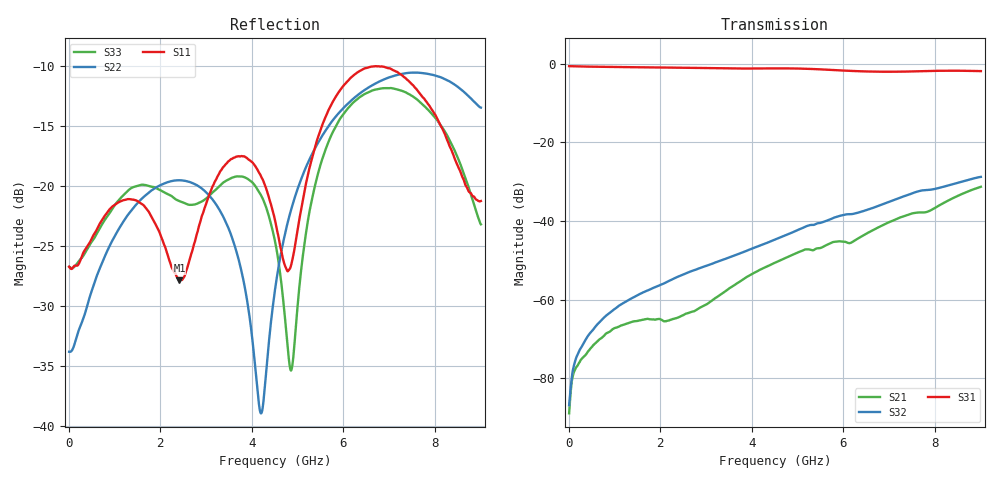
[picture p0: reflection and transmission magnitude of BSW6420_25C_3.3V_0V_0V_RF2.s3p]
!Agilent Technologies,N5230C,MY49001333,A.09.33.09
!Agilent N5230C: A.09.33.09
!Date: Monday, September 23, 2024 13:22:33
!Correction: S11(Full 3 Port(1,2,3))
!S12(Full 3 Port(1,2,3))
!S13(Full 3 Port(1,2,3))
!S21(Full 3 Port(1,2,3))
!S22(Full 3 Port(1,2,3))
!S23(Full 3 Port(1,2,3))
!S31(Full 3 Port(1,2,3))
!S32(Full 3 Port(1,2,3))
!S33(Full 3 Port(1,2,3))
!S3P File: Measurements: <S11,S12,S13>,
!<S21,S22,S23>,
!<S31,S32,S33>:
# Hz S  MA  R 50
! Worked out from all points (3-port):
!   901 points, 10 MHz to 9.01 GHz, reference 50 ohm
!   strongest paths, dB at 10 MHz, 2.26 GHz, 4.51 GHz, 6.76 GHz, 9.01 GHz:
!     S31: -0.6, -1.0, -1.2, -2.0, -1.9
!     S32: -86.8, -54.8, -44.7, -36.2, -28.8
!     S21: -88.9, -64.9, -50.6, -41.7, -31.3
!   lowest |S11| = -27.8 dB at 2.42 GHz (marker M1), VSWR 1.08, Z = 48.2 + j3.56 ohm
!   |S11| at or under -10 dB: start of sweep to end of sweep
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1e7  0.04619 -5.4  3.741e-05 -3.0  0.9313 -2.4
     3.598e-05 -10.0  0.02044 -6.5  3.765e-05 -17.0
     0.9312 -2.3  4.55e-05 1.9  0.04621 -4.4
1e9  0.08343 -155.8  0.0004326 -16.5  0.9095 -102.5
     0.0004347 -16.9  0.06152 -150.8  0.000754 0.5
     0.9101 -102.6  0.000758 1.1  0.08304 -143.7
2.42e9  0.04059 114.6  0.0006034 -99.4  0.888 113.4
        0.0006055 -99.3  0.1058 85.6  0.002021 -106.7
        0.8909 113.6  0.001997 -106.5  0.0867 100.4
3.5e9  0.1272 87.1  0.001382 -149.4  0.8794 3.9
       0.001383 -149.8  0.06638 -1.5  0.003546 164.0
       0.8715 4.0  0.003436 164.1  0.1067 60.1
4.51e9  0.07227 18.5  0.00297 118.1  0.8768 -98.8
        0.002955 118.0  0.03701 127.9  0.005922 76.6
        0.8729 -99.0  0.005808 75.6  0.059 -30.7
5.27e9  0.1204 67.1  0.004362 27.1  0.8628 -176.9
        0.004342 27.1  0.13 56.4  0.00896 3.8
        0.8593 -176.7  0.008878 2.9  0.07954 104.9
6.05e9  0.2673 6.0  0.005433 -60.6  0.8322 103.3
        0.005433 -60.2  0.2157 -7.3  0.01217 -73.2
        0.8165 103.2  0.01213 -74.6  0.2047 22.9
7.11e9  0.3032 -87.8  0.01045 -155.4  0.8024 -4.6
        0.0103 -154.4  0.2879 -95.3  0.01801 -173.7
        0.7917 -6.3  0.0186 -176.2  0.2546 -80.1
8.01e9  0.1987 -159.0  0.01507 127.7  0.8024 -97.3
        0.01472 128.5  0.2887 -173.8  0.02394 92.1
        0.8123 -98.7  0.02565 90.9  0.193 -169.7
9.01e9  0.08674 -178.5  0.02759 37.0  0.7992 157.2
        0.02729 37.2  0.2123 77.7  0.03474 -9.5
        0.8057 157.3  0.03644 -7.8  0.06936 71.2
